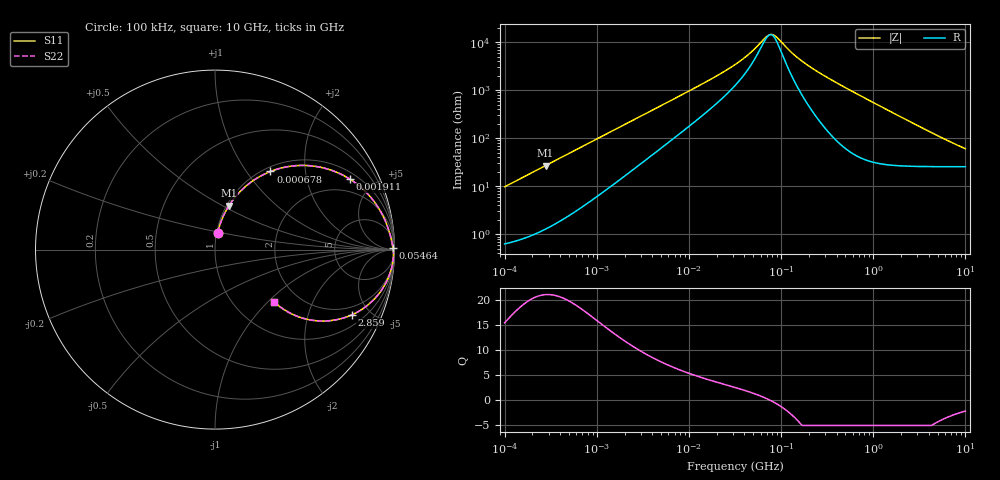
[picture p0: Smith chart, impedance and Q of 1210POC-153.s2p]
# MHz S MA R 50
!Freq  MagS11  AngS11  MagS21  AngS21  MagS12  AngS12  MagS22  AngS22
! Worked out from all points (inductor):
!   801 points, 100 kHz to 10 GHz, reference 50 ohm
!   read as one part in series: L = 15.4 uH near 105.9 kHz
!   highest Q = 21 at 277.8 kHz (marker M1), where L = 15.4 uH
!   self-resonance near 76.02 MHz
!   S11 on the Smith chart (normalised r, x): 100 kHz: 1.01, +0.19; 678 kHz: 1.07, +1.31; 1.911 MHz: 1.30, +3.65; 54.64 MHz: open; 2.859 GHz: 1.52, -3.84; 10 GHz: 1.51, -1.10
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0.1  0.09618 80.8  0.9891 -5.5  0.9891 -5.5  0.09618 80.8
0.2778114  0.2566 72.4  0.9544 -14.8  0.9544 -14.8  0.2566 72.4
0.4403013  0.3845 64.6  0.9043 -22.6  0.9043 -22.6  0.3845 64.6
0.6780317  0.5338 54.6  0.8168 -32.2  0.8168 -32.2  0.5338 54.6
0.6878599  0.539 54.3  0.813 -32.6  0.813 -32.6  0.539 54.3
1.122018  0.7105 41.1  0.6585 -45.1  0.6585 -45.1  0.7105 41.1
1.910953  0.8488 27.5  0.4632 -57.8  0.4632 -57.8  0.8488 27.5
2.900681  0.9121 19.1  0.3286 -65.2  0.3286 -65.2  0.9121 19.1
4.663908  0.9504 12.2  0.2135 -70.5  0.2135 -70.5  0.9504 12.2
10.74608  0.9775 5.4  0.09499 -73.7  0.09499 -73.7  0.9775 5.4
31.62278  0.989 1.6  0.02916 -67.0  0.02916 -67.0  0.989 1.6
42.78091  0.9907 1.0  0.01899 -60.1  0.01899 -60.1  0.9907 1.0
54.63865  0.9918 0.5  0.01231 -48.0  0.01231 -48.0  0.9918 0.5
70.79458  0.9928 0.1  0.007454 -15.1  0.007454 -15.1  0.9928 0.1
82.93732  0.9933 -0.1  0.007084 19.6  0.007084 19.6  0.9933 -0.1
141.2538  0.9946 -1.0  0.01891 72.9  0.01891 72.9  0.9946 -1.0
217.5204  0.9949 -2.0  0.03488 80.6  0.03488 80.6  0.9949 -2.0
613.0558  0.9885 -6.2  0.1088 80.8  0.1088 80.8  0.9885 -6.2
1474.857  0.9486 -14.7  0.2538 71.1  0.2538 71.1  0.9486 -14.7
2859.236  0.8438 -25.6  0.4356 56.7  0.4356 56.7  0.8438 -25.6
5011.872  0.6749 -35.8  0.6003 41.1  0.6003 41.1  0.6749 -35.8
10000  0.4417 -41.5  0.7302 23.6  0.7302 23.6  0.4417 -41.5
